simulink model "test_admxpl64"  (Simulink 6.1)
settings: Solver=ode45  StartTime=0.0  StopTime=250  RelTol=1e-3
undefined symbols (not defined in the file or in its folder): Bit, Location, Lower, netlist, Width
libraries: xbsIndex_r3 x105, adlibrary2 x2

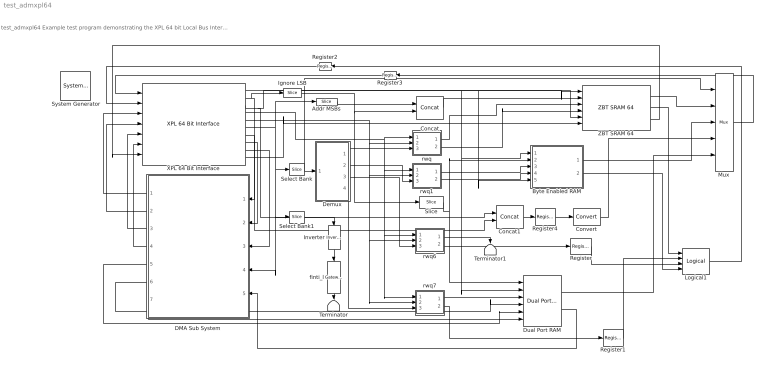
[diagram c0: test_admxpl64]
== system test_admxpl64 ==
  note: test_admxpl64 Example test program demonstrating the XPL 64 bit Local Bus Interface
  " System Generator" : xbsIndex_r3/ System Generator  Tag=genX  xilinxfamily=Virtex2P  part=xc2vp30  speed=-5  package=ff896  synthesis_tool=XST  directory=./netlist  testbench=off  simulink_period=1  sysclk_period=10  incr_netlist=off  trim_vbits=Everywhere in SubSystem  dbl_ovrd=According to Block Masks  core_generation=According to Block Masks  run_coregen=off  deprecated_control=off  eval_field=0
  Addr MSBs : xbsIndex_r3/Slice  mode=Lower Bit Location + Width  nbits=5  bit1=0  base1=MSB of Input  bit0=8  base0=LSB of Input  boolean_output=off  explicit_period=off  period=1  dbl_ovrd=off
  Byte Enabled RAM : Subsystem
  Concat : xbsIndex_r3/Concat  num_inputs=2  explicit_period=off  period=1  dbl_ovrd=off
  Concat1 : xbsIndex_r3/Concat  num_inputs=2  explicit_period=off  period=1  dbl_ovrd=off
  Convert : xbsIndex_r3/Convert  arith_type=Unsigned  n_bits=64  bin_pt=0  quantization=Truncate  overflow=Wrap  latency=0  explicit_period=off  period=1  dbl_ovrd=off  show_param=off  inserted_by_tool=off  pipeline=off
  DMA Sub System : Subsystem  Orientation=left
  Demux : Subsystem
  Dual Port RAM : xbsIndex_r3/Dual Port RAM  depth=1024  initVector=sin(pi*(0:15)/16)  write_mode_A=Read After Write  write_mode_B=Read After Write  latency=1  mem_collision=off  init_zero=on  explicit_period=on  period=1  dbl_ovrd=off  rst_a=off  init_a=0  rst_b=off  init_b=0  show_param=off  distributed_mem=off  use_rpm=off  gen_core=off
  Ignore LSB : xbsIndex_r3/Slice  mode=Lower Bit Location + Width  nbits=15  bit1=0  base1=MSB of Input  bit0=1  base0=LSB of Input  boolean_output=off  explicit_period=off  period=1  dbl_ovrd=off
  Inverter : xbsIndex_r3/Inverter  Orientation=down  latency=0  explicit_period=off  period=1  en=off  dbl_ovrd=off  show_param=off
  Logical1 : xbsIndex_r3/Logical  logical_function=OR  inputs=4  precision=Full  arith_type=Unsigned  n_bits=8  bin_pt=2  align_bp=on  latency=0  explicit_period=off  period=1  en=off  dbl_ovrd=off  show_param=off
  Mux : xbsIndex_r3/Mux  inputs=4  precision=Full  arith_type="Signed  (2's comp)"  n_bits=8  bin_pt=2  quantization=Truncate  overflow=Wrap  latency=0  explicit_period=off  period=1  en=off  dbl_ovrd=off  show_param=off  mux_type=off  use_rpm=off  gen_core=off
  Register : xbsIndex_r3/Register  init=0  reg_only_valid=off  explicit_period=off  period=1  rst=off  en=off  out_en=off  dbl_ovrd=off  show_param=off
  Register1 : xbsIndex_r3/Register  init=0  reg_only_valid=off  explicit_period=off  period=1  rst=off  en=off  out_en=off  dbl_ovrd=off  show_param=off
  Register2 : xbsIndex_r3/Register  Orientation=left  init=0  reg_only_valid=off  explicit_period=on  period=1  rst=off  en=off  out_en=off  dbl_ovrd=off  show_param=off
  Register3 : xbsIndex_r3/Register  Orientation=left  init=0  reg_only_valid=off  explicit_period=on  period=1  rst=off  en=off  out_en=off  dbl_ovrd=off  show_param=off
  Register4 : xbsIndex_r3/Register  init=0  reg_only_valid=off  explicit_period=on  period=1  rst=off  en=off  out_en=off  dbl_ovrd=off  show_param=off
  Select Bank : xbsIndex_r3/Slice  mode=Lower Bit Location + Width  nbits=2  bit1=0  base1=MSB of Input  bit0=0  base0=LSB of Input  boolean_output=off  explicit_period=off  period=1  dbl_ovrd=off
  Select Bank1 : xbsIndex_r3/Slice  mode=Lower Bit Location + Width  nbits=1  bit1=0  base1=MSB of Input  bit0=24  base0=LSB of Input  boolean_output=on  explicit_period=off  period=1  dbl_ovrd=off
  Slice : xbsIndex_r3/Slice  mode=Lower Bit Location + Width  nbits=10  bit1=0  base1=MSB of Input  bit0=0  base0=LSB of Input  boolean_output=off  explicit_period=off  period=1  dbl_ovrd=off
  Terminator : Terminator
  Terminator1 : Terminator
  XPL 64 Bit Interface : adlibrary2/ADM-XPL/XPL 64 Bit Interface  program='load test_admxpl_program.txt'  clock_ratio=1.5
  ZBT SRAM 64 : adlibrary2/ADM-XPL/ZBT SRAM 64
  finti_l : xbsIndex_r3/Gateway Out  Orientation=down  output_type=Double  nbits=8  bin_pt=6  arith_type=Boolean  quantization=Truncate  overflow=Wrap  hdl_port=on  timing_constraint=None  locs_specified=on  LOCs={'G26'}  needs_fixed_name=off  show_param=off
  rwq : Subsystem
  rwq1 : Subsystem
  rwq6 : Subsystem
  rwq7 : Subsystem
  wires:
  XPL 64 Bit Interface/1 -> ZBT SRAM 64/1, Byte Enabled RAM/1(d), Dual Port RAM/2
  Register/1 -> Logical1/3
  Register1/1 -> Logical1/2
  Mux/1 -> Register3/1
  Register2/1 -> XPL 64 Bit Interface/2
  Register3/1 -> XPL 64 Bit Interface/1
  Slice/1 -> Dual Port RAM/1, Byte Enabled RAM/2(a)
  Addr MSBs/1 -> Concat/1
  XPL 64 Bit Interface/2 -> Ignore LSB/1, Concat1/2
  Select Bank/1 -> Demux/1(Select), Mux/1
  rwq6/1(wq) -> Terminator1/1
  rwq6/2(rq) -> Register/1
  rwq7/1(wq) -> Dual Port RAM/3
  rwq7/2(rq) -> Register1/1
  Demux/1(En0) -> rwq/3(e)
  Demux/2(En1) -> rwq1/3(e)
  DMA Sub System/1(Status) -> XPL 64 Bit Interface/3
  DMA Sub System/2(Read IFIFO) -> XPL 64 Bit Interface/4
  DMA Sub System/3(Write OFIFO) -> XPL 64 Bit Interface/5
  DMA Sub System/4(OFIFO_Data) -> XPL 64 Bit Interface/6
  Dual Port RAM/2 -> DMA Sub System/5(DP_RAM_Data)
  DMA Sub System/7(DP_RAM_WE) -> Dual Port RAM/6
  DMA Sub System/6(DP_RAM_Addr) -> Dual Port RAM/4
  DMA Sub System/5(DP_RAM_WData) -> Dual Port RAM/5
  Logical1/1 -> Register2/1
  Select Bank1/1 -> Inverter/1
  Inverter/1 -> finti_l/1
  finti_l/1 -> Terminator/1
  rwq/1(wq) -> ZBT SRAM 64/3
  rwq/2(rq) -> ZBT SRAM 64/4
  Demux/3(En2) -> rwq6/3(e)
  Demux/4(En3) -> rwq7/3(e)
  Register4/1 -> Convert/1
  Dual Port RAM/1 -> Mux/5
  XPL 64 Bit Interface/4 -> rwq/1(w), rwq1/1(w), rwq6/1(w), rwq7/1(w)
  XPL 64 Bit Interface/9 -> DMA Sub System/3(OFIFO_Full)
  XPL 64 Bit Interface/8 -> DMA Sub System/2(IFIFO_Empty)
  XPL 64 Bit Interface/7 -> DMA Sub System/1(IFIFO_Data)
  XPL 64 Bit Interface/6 -> Select Bank/1, DMA Sub System/4(Control), Select Bank1/1, Addr MSBs/1
  XPL 64 Bit Interface/5 -> rwq7/2(r), rwq6/2(r), rwq1/2(r), rwq/2(r)
  Concat/1 -> ZBT SRAM 64/2
  ZBT SRAM 64/2 -> Logical1/1
  Ignore LSB/1 -> Concat/2, Slice/1
  rwq1/1(wq) -> Byte Enabled RAM/3(w)
  Byte Enabled RAM/2(qv) -> Logical1/4
  Byte Enabled RAM/1(q) -> Mux/3
  XPL 64 Bit Interface/3 -> ZBT SRAM 64/5, Byte Enabled RAM/5(be), Concat1/1
  rwq1/2(rq) -> Byte Enabled RAM/4(r)
  Convert/1 -> Mux/4
  Concat1/1 -> Register4/1
  ZBT SRAM 64/1 -> Mux/2
  XPL 64 Bit Interface/10 -> ZBT SRAM 64/6
  ZBT SRAM 64/3 -> XPL 64 Bit Interface/7

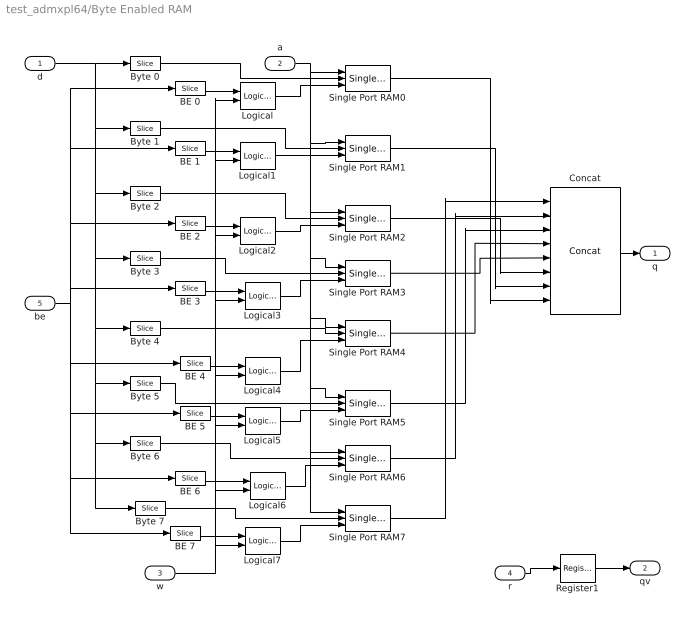
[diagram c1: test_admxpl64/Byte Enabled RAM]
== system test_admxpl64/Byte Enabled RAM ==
  d : Inport  Port=1  LatchInput=off
  a : Inport  Port=2  LatchInput=off
  w : Inport  Port=3  LatchInput=off
  r : Inport  Port=4  LatchInput=off
  be : Inport  Port=5  LatchInput=off
  BE 0 : xbsIndex_r3/Slice  mode=Lower Bit Location + Width  nbits=1  bit1=0  base1=MSB of Input  bit0=0  base0=LSB of Input  boolean_output=on  explicit_period=off  period=1  dbl_ovrd=off
  BE 1 : xbsIndex_r3/Slice  mode=Lower Bit Location + Width  nbits=1  bit1=0  base1=MSB of Input  bit0=1  base0=LSB of Input  boolean_output=on  explicit_period=off  period=1  dbl_ovrd=off
  BE 2 : xbsIndex_r3/Slice  mode=Lower Bit Location + Width  nbits=1  bit1=0  base1=MSB of Input  bit0=2  base0=LSB of Input  boolean_output=on  explicit_period=off  period=1  dbl_ovrd=off
  BE 3 : xbsIndex_r3/Slice  mode=Lower Bit Location + Width  nbits=1  bit1=0  base1=MSB of Input  bit0=3  base0=LSB of Input  boolean_output=on  explicit_period=off  period=1  dbl_ovrd=off
  BE 4 : xbsIndex_r3/Slice  mode=Lower Bit Location + Width  nbits=1  bit1=0  base1=MSB of Input  bit0=4  base0=LSB of Input  boolean_output=on  explicit_period=off  period=1  dbl_ovrd=off
  BE 5 : xbsIndex_r3/Slice  mode=Lower Bit Location + Width  nbits=1  bit1=0  base1=MSB of Input  bit0=5  base0=LSB of Input  boolean_output=on  explicit_period=off  period=1  dbl_ovrd=off
  BE 6 : xbsIndex_r3/Slice  mode=Lower Bit Location + Width  nbits=1  bit1=0  base1=MSB of Input  bit0=6  base0=LSB of Input  boolean_output=on  explicit_period=off  period=1  dbl_ovrd=off
  BE 7 : xbsIndex_r3/Slice  mode=Lower Bit Location + Width  nbits=1  bit1=0  base1=MSB of Input  bit0=7  base0=LSB of Input  boolean_output=on  explicit_period=off  period=1  dbl_ovrd=off
  Byte 0 : xbsIndex_r3/Slice  mode=Lower Bit Location + Width  nbits=8  bit1=0  base1=MSB of Input  bit0=0  base0=LSB of Input  boolean_output=off  explicit_period=off  period=1  dbl_ovrd=off
  Byte 1 : xbsIndex_r3/Slice  mode=Lower Bit Location + Width  nbits=8  bit1=0  base1=MSB of Input  bit0=8  base0=LSB of Input  boolean_output=off  explicit_period=off  period=1  dbl_ovrd=off
  Byte 2 : xbsIndex_r3/Slice  mode=Lower Bit Location + Width  nbits=8  bit1=0  base1=MSB of Input  bit0=16  base0=LSB of Input  boolean_output=off  explicit_period=off  period=1  dbl_ovrd=off
  Byte 3 : xbsIndex_r3/Slice  mode=Lower Bit Location + Width  nbits=8  bit1=0  base1=MSB of Input  bit0=24  base0=LSB of Input  boolean_output=off  explicit_period=off  period=1  dbl_ovrd=off
  Byte 4 : xbsIndex_r3/Slice  mode=Lower Bit Location + Width  nbits=8  bit1=0  base1=MSB of Input  bit0=32  base0=LSB of Input  boolean_output=off  explicit_period=off  period=1  dbl_ovrd=off
  Byte 5 : xbsIndex_r3/Slice  mode=Lower Bit Location + Width  nbits=8  bit1=0  base1=MSB of Input  bit0=40  base0=LSB of Input  boolean_output=off  explicit_period=off  period=1  dbl_ovrd=off
  Byte 6 : xbsIndex_r3/Slice  mode=Lower Bit Location + Width  nbits=8  bit1=0  base1=MSB of Input  bit0=48  base0=LSB of Input  boolean_output=off  explicit_period=off  period=1  dbl_ovrd=off
  Byte 7 : xbsIndex_r3/Slice  mode=Lower Bit Location + Width  nbits=8  bit1=0  base1=MSB of Input  bit0=56  base0=LSB of Input  boolean_output=off  explicit_period=off  period=1  dbl_ovrd=off
  Concat : xbsIndex_r3/Concat  num_inputs=8  explicit_period=off  period=1  dbl_ovrd=off
  Logical{,1..7} (8 alike) : xbsIndex_r3/Logical  logical_function=AND  inputs=2  precision=Full  arith_type=Unsigned  n_bits=8  bin_pt=2  align_bp=on  latency=0  explicit_period=off  period=1  en=off  dbl_ovrd=off  show_param=off
  Register1 : xbsIndex_r3/Register  init=0  reg_only_valid=off  explicit_period=off  period=1  rst=off  en=off  out_en=off  dbl_ovrd=off  show_param=off
  Single Port RAM{0..7} (8 alike) : xbsIndex_r3/Single Port RAM  depth=1024  initVector=sin(pi*(0:15)/16)  write_mode=Read After Write  latency=1  init_zero=on  explicit_period=off  period=1  rst=off  init_reg=0  en=off  dbl_ovrd=off  show_param=off  distributed_mem=off  use_rpm=off  gen_core=off
  q : Outport
  qv : Outport  Port=2
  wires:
  d/1 -> Byte 0/1, Byte 1/1, Byte 2/1, Byte 7/1, Byte 6/1, Byte 5/1, Byte 4/1, Byte 3/1
  be/1 -> BE 7/1, BE 6/1, BE 5/1, BE 0/1, BE 1/1, BE 2/1, BE 4/1, BE 3/1
  BE 0/1 -> Logical/1
  BE 1/1 -> Logical1/1
  BE 2/1 -> Logical2/1
  BE 3/1 -> Logical3/1
  BE 4/1 -> Logical4/1
  BE 5/1 -> Logical5/1
  BE 6/1 -> Logical6/1
  BE 7/1 -> Logical7/1
  w/1 -> Logical7/2, Logical6/2, Logical5/2, Logical4/2, Logical3/2, Logical2/2, Logical1/2, Logical/2
  Logical/1 -> Single Port RAM0/3
  Logical1/1 -> Single Port RAM1/3
  Logical2/1 -> Single Port RAM2/3
  Logical3/1 -> Single Port RAM3/3
  Logical4/1 -> Single Port RAM4/3
  Logical5/1 -> Single Port RAM5/3
  Logical6/1 -> Single Port RAM6/3
  Logical7/1 -> Single Port RAM7/3
  Byte 7/1 -> Single Port RAM7/2
  Byte 6/1 -> Single Port RAM6/2
  Byte 5/1 -> Single Port RAM5/2
  Byte 4/1 -> Single Port RAM4/2
  Byte 3/1 -> Single Port RAM3/2
  Byte 2/1 -> Single Port RAM2/2
  Byte 1/1 -> Single Port RAM1/2
  Byte 0/1 -> Single Port RAM0/2
  a/1 -> Single Port RAM0/1, Single Port RAM7/1, Single Port RAM6/1, Single Port RAM5/1, Single Port RAM4/1, Single Port RAM3/1, Single Port RAM2/1, Single Port RAM1/1
  r/1 -> Register1/1
  Register1/1 -> qv/1
  Single Port RAM7/1 -> Concat/1
  Single Port RAM6/1 -> Concat/2
  Single Port RAM5/1 -> Concat/3
  Single Port RAM4/1 -> Concat/4
  Single Port RAM3/1 -> Concat/5
  Single Port RAM2/1 -> Concat/6
  Single Port RAM1/1 -> Concat/7
  Single Port RAM0/1 -> Concat/8
  Concat/1 -> q/1

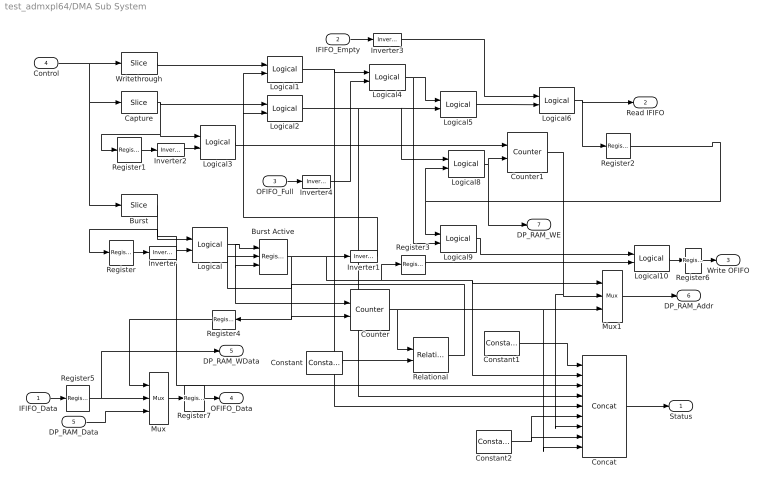
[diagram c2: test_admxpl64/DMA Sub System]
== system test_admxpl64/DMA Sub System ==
  IFIFO_Data : Inport  Port=1  LatchInput=off
  IFIFO_Empty : Inport  Port=2  LatchInput=off
  OFIFO_Full : Inport  Port=3  LatchInput=off
  Control : Inport  Port=4  LatchInput=off
  DP_RAM_Data : Inport  Port=5  LatchInput=off
  Burst : xbsIndex_r3/Slice  mode=Lower Bit Location + Width  nbits=1  bit1=0  base1=MSB of Input  bit0=18  base0=LSB of Input  boolean_output=on  explicit_period=on  period=1  dbl_ovrd=off
  Burst Active : xbsIndex_r3/Register  init=0  reg_only_valid=off  explicit_period=on  period=1  rst=on  en=on  out_en=off  dbl_ovrd=off  show_param=off
  Capture : xbsIndex_r3/Slice  mode=Lower Bit Location + Width  nbits=1  bit1=0  base1=MSB of Input  bit0=17  base0=LSB of Input  boolean_output=on  explicit_period=on  period=1  dbl_ovrd=off
  Concat : xbsIndex_r3/Concat  num_inputs=9  explicit_period=on  period=1  dbl_ovrd=off
  Constant : xbsIndex_r3/Constant  const=511  equ=P=C  arith_type=Unsigned  n_bits=10  bin_pt=0  opselect=C  inp2=PCIN>>17  opr=+  inp1=P  carry=CIN  iostate=0  explicit_period=off  period=1  dbl_ovrd=off
  Constant1 : xbsIndex_r3/Constant  const=0  equ=P=C  arith_type=Unsigned  n_bits=36  bin_pt=0  opselect=C  inp2=PCIN>>17  opr=+  inp1=P  carry=CIN  iostate=0  explicit_period=off  period=1  dbl_ovrd=off
  Constant2 : xbsIndex_r3/Constant  const=0  equ=P=C  arith_type=Unsigned  n_bits=2  bin_pt=0  opselect=C  inp2=PCIN>>17  opr=+  inp1=P  carry=CIN  iostate=0  explicit_period=off  period=1  dbl_ovrd=off
  Counter : xbsIndex_r3/Counter  cnt_type=Count Limited  n_bits=10  bin_pt=0  arith_type=Unsigned  start_count=0  cnt_to=Inf  cnt_by_val=1  operation=Up  explicit_period=on  period=1  load_pin=off  rst=on  en=on  dbl_ovrd=off  show_param=off  use_rpm=on  gen_core=off
  Counter1 : xbsIndex_r3/Counter  cnt_type=Count Limited  n_bits=10  bin_pt=0  arith_type=Unsigned  start_count=0  cnt_to=Inf  cnt_by_val=1  operation=Up  explicit_period=on  period=1  load_pin=off  rst=on  en=on  dbl_ovrd=off  show_param=off  use_rpm=on  gen_core=off
  Inverter{,1..2,4} (4 alike) : xbsIndex_r3/Inverter  latency=0  explicit_period=off  period=1  en=off  dbl_ovrd=off  show_param=off
  Inverter3 : xbsIndex_r3/Inverter  latency=0  explicit_period=on  period=1  en=off  dbl_ovrd=off  show_param=off
  Logical : xbsIndex_r3/Logical  logical_function=AND  inputs=2  precision=Full  arith_type=Unsigned  n_bits=8  bin_pt=2  align_bp=on  latency=0  explicit_period=on  period=1  en=off  dbl_ovrd=off  show_param=off
  Logical{1..2,4,8..9} (5 alike) : xbsIndex_r3/Logical  logical_function=AND  inputs=2  precision=Full  arith_type=Unsigned  n_bits=8  bin_pt=2  align_bp=on  latency=0  explicit_period=off  period=1  en=off  dbl_ovrd=off  show_param=off
  Logical10 : xbsIndex_r3/Logical  logical_function=OR  inputs=2  precision=Full  arith_type=Unsigned  n_bits=8  bin_pt=2  align_bp=on  latency=0  explicit_period=on  period=1  en=off  dbl_ovrd=off  show_param=off
  Logical3 : xbsIndex_r3/Logical  logical_function=AND  inputs=2  precision=Full  arith_type=Unsigned  n_bits=8  bin_pt=2  align_bp=on  latency=0  explicit_period=on  period=1  en=off  dbl_ovrd=off  show_param=off
  Logical5 : xbsIndex_r3/Logical  logical_function=OR  inputs=2  precision=Full  arith_type=Unsigned  n_bits=8  bin_pt=2  align_bp=on  latency=0  explicit_period=off  period=1  en=off  dbl_ovrd=off  show_param=off
  Logical6 : xbsIndex_r3/Logical  logical_function=AND  inputs=2  precision=Full  arith_type=Unsigned  n_bits=8  bin_pt=2  align_bp=on  latency=0  explicit_period=on  period=1  en=off  dbl_ovrd=off  show_param=off
  Mux : xbsIndex_r3/Mux  inputs=2  precision=Full  arith_type="Signed  (2's comp)"  n_bits=8  bin_pt=2  quantization=Truncate  overflow=Wrap  latency=0  explicit_period=on  period=1  en=off  dbl_ovrd=off  show_param=off  mux_type=off  use_rpm=off  gen_core=off
  Mux1 : xbsIndex_r3/Mux  inputs=2  precision=Full  arith_type="Signed  (2's comp)"  n_bits=8  bin_pt=2  quantization=Truncate  overflow=Wrap  latency=0  explicit_period=off  period=1  en=off  dbl_ovrd=off  show_param=off  mux_type=off  use_rpm=off  gen_core=off
  Register{,1..3,5..7} (7 alike) : xbsIndex_r3/Register  init=0  reg_only_valid=off  explicit_period=on  period=1  rst=off  en=off  out_en=off  dbl_ovrd=off  show_param=off
  Register4 : xbsIndex_r3/Register  Orientation=left  init=0  reg_only_valid=off  explicit_period=on  period=1  rst=off  en=off  out_en=off  dbl_ovrd=off  show_param=off
  Relational : xbsIndex_r3/Relational  mode=a=b  latency=0  explicit_period=off  period=1  en=off  dbl_ovrd=off  show_param=off
  Writethrough : xbsIndex_r3/Slice  mode=Lower Bit Location + Width  nbits=1  bit1=0  base1=MSB of Input  bit0=16  base0=LSB of Input  boolean_output=on  explicit_period=on  period=1  dbl_ovrd=off
  Status : Outport
  Read IFIFO : Outport  Port=2
  Write OFIFO : Outport  Port=3
  OFIFO_Data : Outport  Port=4
  DP_RAM_WData : Outport  Port=5
  DP_RAM_Addr : Outport  Port=6
  DP_RAM_WE : Outport  Port=7
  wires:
  Mux/1 -> Register7/1
  IFIFO_Data/1 -> Register5/1
  DP_RAM_Data/1 -> Mux/3
  Control/1 -> Writethrough/1, Burst/1, Capture/1
  Burst/1 -> Register/1, Logical/1, Concat/3
  Register/1 -> Inverter/1
  Inverter/1 -> Logical/2
  Logical/1 -> Burst Active/1, Burst Active/3, Counter/1
  Burst Active/1 -> Inverter1/1, Register3/1, Mux1/1, Concat/2, Counter/2, Register4/1
  Inverter1/1 -> Logical1/2, Logical2/2
  Capture/1 -> Logical2/1, Logical3/1, Register1/1
  Writethrough/1 -> Logical1/1
  Register1/1 -> Inverter2/1
  Inverter2/1 -> Logical3/2
  Logical3/1 -> Counter1/1
  IFIFO_Empty/1 -> Inverter3/1
  OFIFO_Full/1 -> Inverter4/1
  Logical1/1 -> Logical4/1, Concat/5
  Inverter4/1 -> Logical4/2
  Logical2/1 -> Logical5/2, Logical8/1, Concat/4
  Logical4/1 -> Logical5/1, Logical9/2
  Inverter3/1 -> Logical6/1
  Logical5/1 -> Logical6/2
  Logical6/1 -> Read IFIFO/1, Register2/1
  Register2/1 -> Logical8/2, Logical9/1
  Logical8/1 -> Counter1/2, DP_RAM_WE/1
  Mux1/1 -> DP_RAM_Addr/1
  Counter1/1 -> Mux1/2, Concat/7
  Counter/1 -> Relational/1, Mux1/3, Concat/9
  Logical9/1 -> Logical10/1
  Register3/1 -> Logical10/2
  Constant/1 -> Relational/2
  Relational/1 -> Burst Active/2
  Constant2/1 -> Concat/8, Concat/6
  Concat/1 -> Status/1
  Constant1/1 -> Concat/1
  Logical10/1 -> Register6/1
  Register4/1 -> Mux/1
  Register5/1 -> Mux/2, DP_RAM_WData/1
  Register6/1 -> Write OFIFO/1
  Register7/1 -> OFIFO_Data/1

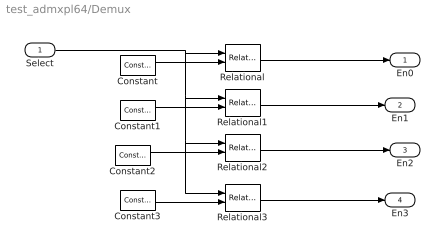
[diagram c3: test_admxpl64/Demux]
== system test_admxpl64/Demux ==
  Select : Inport  Port=1  LatchInput=off
  Constant : xbsIndex_r3/Constant  const=0  equ=P=C  arith_type=Unsigned  n_bits=2  bin_pt=0  opselect=C  inp2=PCIN>>17  opr=+  inp1=P  carry=CIN  iostate=0  explicit_period=off  period=1  dbl_ovrd=off
  Constant1 : xbsIndex_r3/Constant  const=1  equ=P=C  arith_type=Unsigned  n_bits=2  bin_pt=0  opselect=C  inp2=PCIN>>17  opr=+  inp1=P  carry=CIN  iostate=0  explicit_period=off  period=1  dbl_ovrd=off
  Constant2 : xbsIndex_r3/Constant  const=2  equ=P=C  arith_type=Unsigned  n_bits=2  bin_pt=0  opselect=C  inp2=PCIN>>17  opr=+  inp1=P  carry=CIN  iostate=0  explicit_period=off  period=1  dbl_ovrd=off
  Constant3 : xbsIndex_r3/Constant  const=3  equ=P=C  arith_type=Unsigned  n_bits=2  bin_pt=0  opselect=C  inp2=PCIN>>17  opr=+  inp1=P  carry=CIN  iostate=0  explicit_period=off  period=1  dbl_ovrd=off
  Relational{,1..3} (4 alike) : xbsIndex_r3/Relational  mode=a=b  latency=0  explicit_period=off  period=1  en=off  dbl_ovrd=off  show_param=off
  En0 : Outport
  En1 : Outport  Port=2
  En2 : Outport  Port=3
  En3 : Outport  Port=4
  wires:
  Relational/1 -> En0/1
  Relational1/1 -> En1/1
  Relational2/1 -> En2/1
  Relational3/1 -> En3/1
  Select/1 -> Relational/1, Relational1/1, Relational2/1, Relational3/1
  Constant/1 -> Relational/2
  Constant1/1 -> Relational1/2
  Constant2/1 -> Relational2/2
  Constant3/1 -> Relational3/2

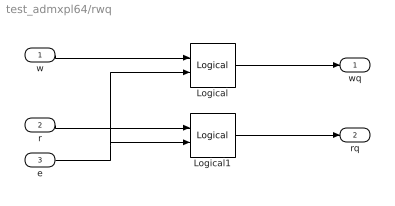
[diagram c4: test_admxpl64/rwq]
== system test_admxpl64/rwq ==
  w : Inport  Port=1  LatchInput=off
  r : Inport  Port=2  LatchInput=off
  e : Inport  Port=3  LatchInput=off
  Logical : xbsIndex_r3/Logical  logical_function=AND  inputs=2  precision=Full  arith_type=Unsigned  n_bits=8  bin_pt=2  align_bp=on  latency=0  explicit_period=off  period=1  en=off  dbl_ovrd=off  show_param=off
  Logical1 : xbsIndex_r3/Logical  logical_function=AND  inputs=2  precision=Full  arith_type=Unsigned  n_bits=8  bin_pt=2  align_bp=on  latency=0  explicit_period=off  period=1  en=off  dbl_ovrd=off  show_param=off
  wq : Outport
  rq : Outport  Port=2
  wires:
  e/1 -> Logical1/2, Logical/2
  r/1 -> Logical1/1
  w/1 -> Logical/1
  Logical/1 -> wq/1
  Logical1/1 -> rq/1

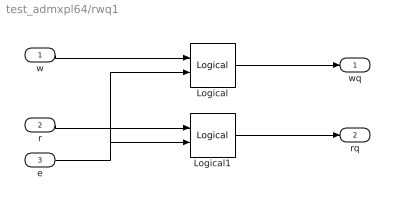
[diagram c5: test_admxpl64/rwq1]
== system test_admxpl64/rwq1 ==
  w : Inport  Port=1  LatchInput=off
  r : Inport  Port=2  LatchInput=off
  e : Inport  Port=3  LatchInput=off
  Logical : xbsIndex_r3/Logical  logical_function=AND  inputs=2  precision=Full  arith_type=Unsigned  n_bits=8  bin_pt=2  align_bp=on  latency=0  explicit_period=off  period=1  en=off  dbl_ovrd=off  show_param=off
  Logical1 : xbsIndex_r3/Logical  logical_function=AND  inputs=2  precision=Full  arith_type=Unsigned  n_bits=8  bin_pt=2  align_bp=on  latency=0  explicit_period=off  period=1  en=off  dbl_ovrd=off  show_param=off
  wq : Outport
  rq : Outport  Port=2
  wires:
  e/1 -> Logical1/2, Logical/2
  r/1 -> Logical1/1
  w/1 -> Logical/1
  Logical/1 -> wq/1
  Logical1/1 -> rq/1

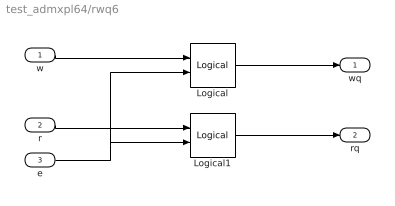
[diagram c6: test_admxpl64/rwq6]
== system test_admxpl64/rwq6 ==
  w : Inport  Port=1  LatchInput=off
  r : Inport  Port=2  LatchInput=off
  e : Inport  Port=3  LatchInput=off
  Logical : xbsIndex_r3/Logical  logical_function=AND  inputs=2  precision=Full  arith_type=Unsigned  n_bits=8  bin_pt=2  align_bp=on  latency=0  explicit_period=off  period=1  en=off  dbl_ovrd=off  show_param=off
  Logical1 : xbsIndex_r3/Logical  logical_function=AND  inputs=2  precision=Full  arith_type=Unsigned  n_bits=8  bin_pt=2  align_bp=on  latency=0  explicit_period=off  period=1  en=off  dbl_ovrd=off  show_param=off
  wq : Outport
  rq : Outport  Port=2
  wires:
  e/1 -> Logical1/2, Logical/2
  r/1 -> Logical1/1
  w/1 -> Logical/1
  Logical/1 -> wq/1
  Logical1/1 -> rq/1

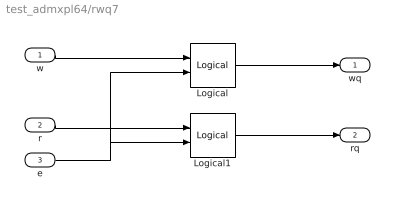
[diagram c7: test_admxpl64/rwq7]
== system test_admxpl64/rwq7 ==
  w : Inport  Port=1  LatchInput=off
  r : Inport  Port=2  LatchInput=off
  e : Inport  Port=3  LatchInput=off
  Logical : xbsIndex_r3/Logical  logical_function=AND  inputs=2  precision=Full  arith_type=Unsigned  n_bits=8  bin_pt=2  align_bp=on  latency=0  explicit_period=off  period=1  en=off  dbl_ovrd=off  show_param=off
  Logical1 : xbsIndex_r3/Logical  logical_function=AND  inputs=2  precision=Full  arith_type=Unsigned  n_bits=8  bin_pt=2  align_bp=on  latency=0  explicit_period=off  period=1  en=off  dbl_ovrd=off  show_param=off
  wq : Outport
  rq : Outport  Port=2
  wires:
  e/1 -> Logical1/2, Logical/2
  r/1 -> Logical1/1
  w/1 -> Logical/1
  Logical/1 -> wq/1
  Logical1/1 -> rq/1
